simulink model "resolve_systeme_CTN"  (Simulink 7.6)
settings: Solver=ode45  StartTime=0.0  StopTime=10.0  RelTol=1e-3

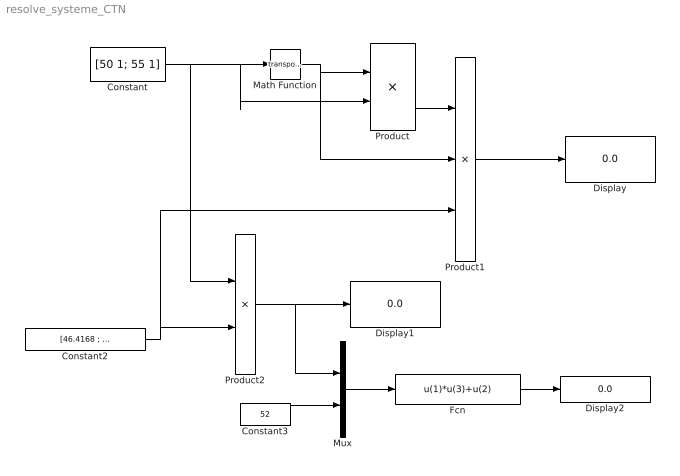
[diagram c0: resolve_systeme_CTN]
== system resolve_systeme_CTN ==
  Constant : Constant  Value=[50 1; 55 1]  VectorParams1D=off
  Constant2 : Constant  Value=[46.4168 ; 46.4286]
  Constant3 : Constant  Value=52
  Display : Display
  Display1 : Display
  Display2 : Display
  Fcn : Fcn  Expr=u(1)*u(3)+u(2)
  Math Function : Math  Operator=transpose
  Mux : Mux  Inputs=2
  Product : Product  Multiplication=Matrix(*)
  Product1 : Product  Inputs=/**  Multiplication=Matrix(*)
  Product2 : Product  Inputs=/*  Multiplication=Matrix(*)
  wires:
  Constant/1 -> Math Function/1, Product/2, Product2/1
  Math Function/1 -> Product/1, Product1/2
  Product/1 -> Product1/1
  Product1/1 -> Display/1
  Constant2/1 -> Product2/2, Product1/3
  Product2/1 -> Display1/1, Mux/1
  Constant3/1 -> Mux/2
  Mux/1 -> Fcn/1
  Fcn/1 -> Display2/1
